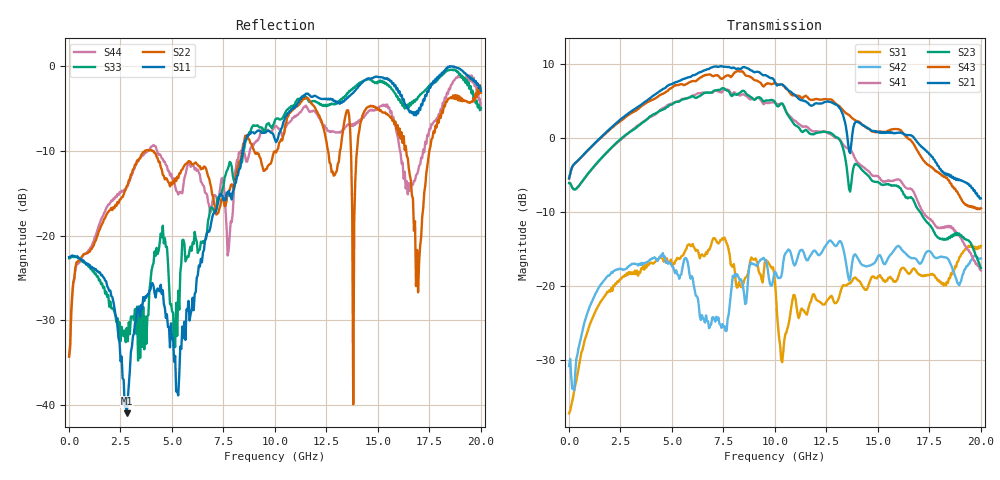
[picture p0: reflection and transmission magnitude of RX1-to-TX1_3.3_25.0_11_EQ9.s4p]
!Agilent Technologies,N5225A,MY51451112,A.09.50.13
!Agilent N5225A: A.09.50.13
!Date: Wednesday, January 31, 2018 11:04:45
!Correction: S11(Full 4 Port(1,2,3,4))
!S12(Full 4 Port(1,2,3,4))
!S13(Full 4 Port(1,2,3,4))
!S14(Full 4 Port(1,2,3,4))
!S21(Full 4 Port(1,2,3,4))
!S22(Full 4 Port(1,2,3,4))
!S23(Full 4 Port(1,2,3,4))
!S24(Full 4 Port(1,2,3,4))
!S31(Full 4 Port(1,2,3,4))
!S32(Full 4 Port(1,2,3,4))
!S33(Full 4 Port(1,2,3,4))
!S34(Full 4 Port(1,2,3,4))
!S41(Full 4 Port(1,2,3,4))
!S42(Full 4 Port(1,2,3,4))
!S43(Full 4 Port(1,2,3,4))
!S44(Full 4 Port(1,2,3,4))
!S4P File: Measurements: <S11,S12,S13,S14>,
!<S21,S22,S23,S24>,
!<S31,S32,S33,S34>,
!<S41,S42,S43,S44>:
# Hz S  RI  R 50
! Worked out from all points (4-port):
!   401 points, 10 MHz to 20 GHz, reference 50 ohm
!   strongest paths, dB at 10 MHz, 5.008 GHz, 10.01 GHz, 15 GHz, 20 GHz:
!     S21: -5.4, 7.3, 7.6, 0.9, -8.1
!     S43: -5.5, 6.8, 7.5, 0.9, -9.5
!     S23: -6.1, 4.5, 4.9, -5.9, -17.5
!     S41: -6.1, 4.7, 4.8, -5.1, -17.8
!     S42: -30.8, -17.3, -18.0, -16.0, -16.2
!     S31: -37.1, -17.2, -19.4, -18.7, -14.6
!   lowest |S11| = -41.0 dB at 2.809 GHz (marker M1), VSWR 1.02, Z = 49.7 - j0.846 ohm
!   |S11| at or under -10 dB: start of sweep to 8.442 GHz
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1e7  -0.0745 -0.00279  -0.000484 0.000676  0.0141 0.000453  0.000226 0.000563
     0.5361 0.0112  -0.0131 0.0141  -0.4977 0.000154  0.0264 0.012
     0.0139 0.00064  0.000199 0.000532  -0.0733 -0.00414  -0.000147 0.000379
     -0.4978 0.000695  0.0261 0.0126  0.5336 0.0103  -0.0127 0.0148
2.8086e9  -0.00263 -0.0085  0.0166 0.00259  0.0546 0.1092  0.018 0.000204
          1.133 -0.8918  0.1958 0.00289  -0.7898 0.7139  0.1029 0.0917
          0.0597 0.1066  0.0198 0.00319  0.0154 0.0239  0.0216 0.0004
          -0.68 0.8129  0.0911 0.0956  0.8907 -1.092  0.1873 -0.0497
7.0065e9  -0.0311 0.1308  0.0143 -0.0157  0.1351 0.0709  0.0088 -0.0306
          -3.023 0.1319  0.1079 -0.1293  2.025 -0.4205  0.0385 0.0256
          0.1624 0.1343  0.0234 -0.016  0.0241 0.1426  0.0223 -0.0361
          1.666 -1.189  0.0613 -0.00855  -2.231 1.376  0.0924 -0.1433
8.655675e9  -0.00612 0.3879  0.00347 -0.00865  0.0792 0.0695  -0.00786 -0.0177
            -0.8266 2.845  -0.1162 0.3739  0.1986 -1.954  -0.00695 0.1304
            0.0972 0.0667  0.00919 -0.0206  0.031 0.3881  -0.0119 -0.0296
            -0.7 -1.77  -0.0282 0.088  0.7087 2.536  0.1993 0.1867
1.050475e10  0.154 0.4794  -0.0284 -0.0333  0.0133 0.017  -0.0486 -0.00313
             1.859 1.197  0.3054 0.3298  -1.482 -0.4559  0.0532 0.1882
             -0.0189 0.0434  -0.0362 -0.0301  0.2225 0.4856  -0.0537 -0.0086
             -1.515 0.3652  0.0816 0.1449  2.179 -0.0732  0.4198 -0.1067
1.42029e10  0.6698 0.4232  -0.0285 0.000333  0.00522 0.092  -0.0122 0.0128
            0.274 -1.21  0.4575 0.1494  0.0399 0.615  0.1503 0.0358
            0.0152 0.102  -0.0134 -0.00147  0.7638 0.2691  -0.0229 0.0173
            0.5349 0.3728  0.1289 0.056  -0.9775 -0.7731  -0.1527 -0.4603
2e10  0.7122 0.0684  0.0231 0.0348  -0.0793 0.1616  0.0347 0.0209
      0.0115 0.3917  0.6934 0.0748  0.0158 -0.1321  0.1537 0.0409
      -0.0791 0.1694  0.00631 0.0477  0.5645 -0.026  0.0475 0.0206
      -0.1171 -0.052  0.1473 0.046  0.3166 0.114  -0.1521 -0.5317
